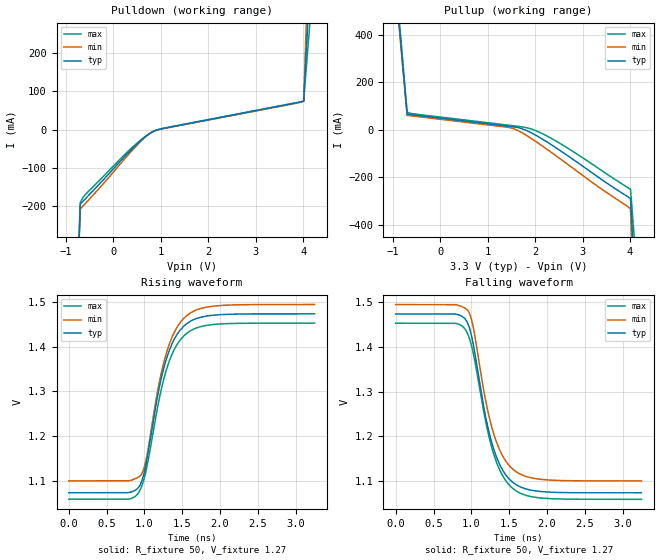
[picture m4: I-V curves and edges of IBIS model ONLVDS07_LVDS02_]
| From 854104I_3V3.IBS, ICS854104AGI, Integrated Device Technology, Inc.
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[Model]   ONLVDS07_LVDS02_
Model_type   Output
Polarity   Non-Inverting
|   typ   min   max
C_comp   2pF   1.5pF   2.5pF
Vmeas = 1.27V
Rref = 50
Cref = 0
Vref = 1.27V
|   typ   min   max
[Voltage range]   3.3V   3.135V   3.465V
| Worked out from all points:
|   slope of the pulldown table from 0 to 0.495 V, typ, clamps not added: 7.72 ohm
|   slope of the pullup table from 0 to 0.495 V, typ, clamps not added: 42.1 ohm
|   rising waveform, R_fixture 50, V_fixture 1.27: 20-80 % time 294ps typ, 295ps min, 303ps max; typ from 1.07 V to 1.47 V
|   falling waveform, R_fixture 50, V_fixture 1.27: 20-80 % time 294ps typ, 295ps min, 303ps max; typ from 1.47 V to 1.07 V
[Pulldown]
|Voltage   I (typ)   I (min)   I (max)
-3.3V     -12.65A    -15.46A    -10.98A
-1.22V    -2.111A    -2.068A    -2.153A
-700mV    -193.8mA   -206.5mA   -190.5mA
-645mV    -186.6mA   -199.2mA   -176.4mA
-591mV    -179.6mA   -192mA     -168.6mA
381.2mV   -51.39mA   -55.77mA   -47.77mA
651.3mV   -20.4mA    -21.4mA    -19.48mA
813.3mV   -6.203mA   -5.872mA   -6.355mA
1.083V    4.273mA    3.578mA    4.591mA
4.01V     74.38mA    74.89mA    74.44mA
4.528V    1.282A     1.92A      877.3mA
6.6V      7.966A     10.44A     6.456A
[Pullup]
|Voltage   I (typ)   I (min)   I (max)
-3.3V     7.958A     9.751A     6.893A
-1.22V    1.248A     1.203A     1.29A
-700mV    66.02mA    60.62mA    74.84mA
-537mV    61.66mA    56.73mA    66.33mA
1.461V    14.18mA    8.952mA    18.64mA
1.623V    9.51mA     -2.335mA   14.76mA
1.786V    -533.3uA   -20.17mA   10.05mA
2.164V    -40.74mA   -70.36mA   -17.8mA
2.704V    -111.8mA   -148.4mA   -79.91mA
4.01V     -290.1mA   -334mA     -250.7mA
4.528V    -2.246A    -3.273A    -1.583A
6.6V      -12.68A    -16.56A    -10.3A
[Ramp]
|   typ   min   max
dV/dt_r   0.321/0.466n   0.316/0.465n   0.316/0.481n
dV/dt_f   0.321/0.466n   0.316/0.465n   0.316/0.481n
R_load =   50.0000
[Rising Waveform]
R_fixture = 50
V_fixture = 1.27   |Vcc_typ
V_fixture_min = 1.285 |Vcc_min
V_fixture_max = 1.26  |Vcc_max
C_fixture = 0.0p
| Time   typ   min   max
0s        1.073V     1.099V     1.058V
793.8ps   1.073V     1.1V       1.059V
956.5ps   1.095V     1.113V     1.084V
1.025ns   1.14V      1.149V     1.125V
1.171ns   1.288V     1.298V     1.262V
1.275ns   1.364V     1.377V     1.34V
1.405ns   1.42V      1.436V     1.397V
1.565ns   1.453V     1.471V     1.431V
1.965ns   1.472V     1.492V     1.451V
3.25ns    1.474V     1.495V     1.453V
[Falling Waveform]
R_fixture = 50
V_fixture = 1.27   |Vcc_typ
V_fixture_min = 1.285 |Vcc_min
V_fixture_max = 1.26  |Vcc_max
C_fixture = 0.0p
| Time   typ   min   max
0s        1.474V     1.495V     1.453V
793.8ps   1.474V     1.495V     1.453V
956.5ps   1.451V     1.481V     1.427V
1.025ns   1.407V     1.445V     1.387V
1.171ns   1.259V     1.296V     1.249V
1.275ns   1.183V     1.217V     1.172V
1.405ns   1.126V     1.158V     1.114V
1.565ns   1.094V     1.124V     1.08V
1.965ns   1.075V     1.102V     1.061V
3.25ns    1.073V     1.099V     1.058V
